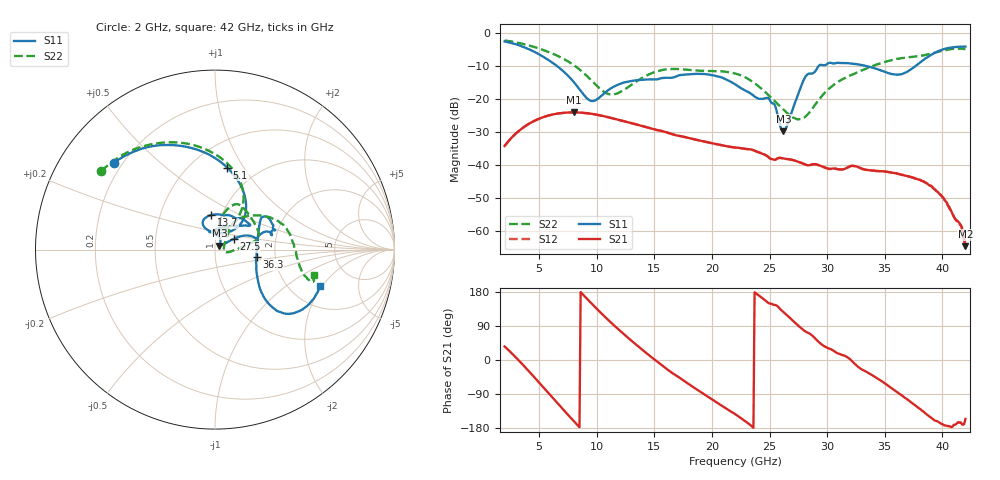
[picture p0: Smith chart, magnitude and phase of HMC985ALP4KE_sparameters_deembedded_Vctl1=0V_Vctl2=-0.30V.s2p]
!s2p File: Measurements: S11, S21, S12, S22
# GHz S dB R 50.0
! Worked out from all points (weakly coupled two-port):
!   401 points, 2 GHz to 42 GHz, reference 50 ohm
!   highest |S21| = -24.11 dB at 8 GHz (marker M1); lowest = -64.7 dB at 42 GHz (marker M2)
!   lowest |S11| = -29.8 dB at 26.2 GHz (marker M3), VSWR 1.07, Z = 52.5 + j2.22 ohm
!   |S11| at or under -10 dB: 6.53 GHz to 29.27 GHz (22.74 GHz wide, 127 % of centre); 33.34 GHz to 37.69 GHz (4.35 GHz wide, 12.2 % of centre)
!   |S22| runs from -26.2 to -2.3 dB; largest |S21 - S12| = 0.00017
!   S11 on the Smith chart (normalised r, x): 2 GHz: 0.17, +0.36; 5.1 GHz: 0.73, +0.85; 13.7 GHz: 0.89, +0.35; 27.5 GHz: 1.22, +0.15; 36.3 GHz: 1.59, -0.14; 42 GHz: 2.91, -1.91
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2  -2.58 139.5  -34.31 35.7  -34.33 35.8  -2.28 145.4
3.5  -4.07 111.6  -29.02 -9.8  -29.03 -9.8  -3.26 121.6
5.1  -6.70 81.6  -25.89 -63.1  -25.89 -63.1  -4.87 97.2
8  -14.87 45.0  -24.11 -161.2  -24.12 -161.2  -9.75 60.7
8.7  -18.03 51.5  -24.21 176.0  -24.21 176.0  -11.66 56.0
9.7  -20.66 87.0  -24.63 144.4  -24.63 144.4  -14.98 54.7
11.2  -16.89 115.7  -25.77 99.7  -25.77 99.7  -18.66 70.4
13.7  -14.29 96.7  -28.03 33.3  -28.04 33.3  -14.14 77.5
15.4  -13.94 73.0  -29.57 -7.6  -29.58 -7.6  -11.48 68.3
19.4  -12.51 34.7  -33.03 -91.9  -33.03 -92.0  -11.53 34.6
22  -15.57 52.2  -34.78 -142.6  -34.78 -142.7  -12.31 14.1
25  -20.23 97.6  -38.01 149.1  -38.04 149.1  -19.22 -1.6
26.2  -29.82 40.8  -38.08 126.5  -38.09 126.4  -23.28 -12.7
27.5  -18.42 29.6  -39.12 90.0  -39.14 90.0  -26.18 -1.0
28.1  -13.37 20.7  -39.96 75.5  -39.93 75.5  -25.45 19.4
28.7  -12.32 12.8  -39.93 64.6  -39.92 64.5  -23.01 36.3
31.1  -9.13 24.1  -41.43 15.4  -41.44 15.4  -14.52 55.0
35.4  -12.27 12.4  -42.28 -70.1  -42.29 -70.4  -8.45 25.7
36.3  -12.57 -10.1  -42.89 -89.7  -42.85 -89.6  -7.77 17.9
39.8  -5.31 -41.3  -49.06 -166.0  -48.98 -166.3  -5.55 -16.6
41.5  -4.18 -23.0  -57.77 -165.4  -58.08 -162.6  -4.75 -17.4
42  -4.14 -19.0  -64.73 -155.5  -64.39 -160.0  -4.90 -14.5
